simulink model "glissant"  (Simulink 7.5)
settings: Solver=ode45  StartTime=0.0  StopTime=10  RelTol=1e-3

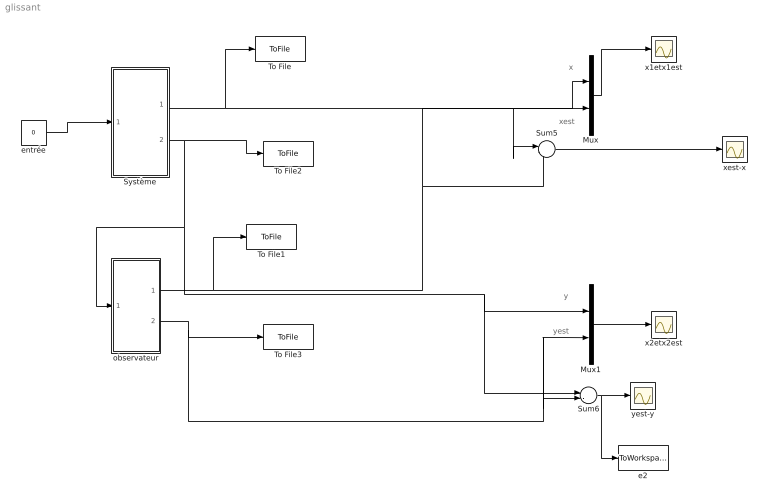
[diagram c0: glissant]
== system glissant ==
  note: x
  note: xest
  note: y
  note: yest
  Mux : Mux  Inputs=2
  Mux1 : Mux  Inputs=2
  Sum5 : Sum  Inputs=|-+  OutDataType=sfix(16)  OutScaling=2^0
  Sum6 : Sum  Inputs=|-+  OutDataType=sfix(16)  OutScaling=2^0
  Système : Subsystem
  To File : ToFile  Filename=x1.mat
  To File1 : ToFile  Filename=x1est.mat
  To File2 : ToFile  Filename=x2.mat
  To File3 : ToFile  Filename=x2est.mat
  e2 : ToWorkspace  VariableName=y  SampleTime=-1  SaveFormat=Array
  entrée : Constant  Value=0  OutDataType=fixdt(1, 16)  OutScaling=2^0
  observateur : Subsystem
  x1etx1est : Scope
  x2etx2est : Scope
  xest-x : Scope
  yest-y : Scope
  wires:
  Mux/1 -> x1etx1est/1
  Sum6/1 -> yest-y/1, e2/1
  Sum5/1 -> xest-x/1
  entrée/1 -> Système/1(u)
  Système/1("x1 ") -> Mux/1, Sum5/1, To File/1
  Système/2("x2 ") -> observateur/1(y), Mux1/1, Sum6/1, To File2/1
  observateur/1("x1 ") -> Sum5/2, Mux/2, To File1/1
  observateur/2("yest ") -> Sum6/2, Mux1/2, To File3/1
  Mux1/1 -> x2etx2est/1

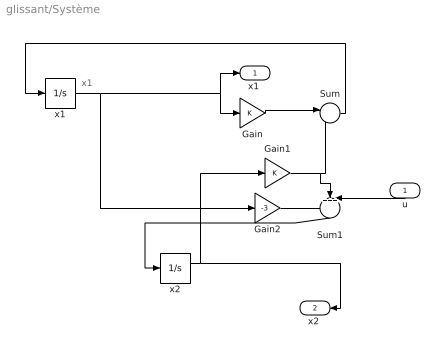
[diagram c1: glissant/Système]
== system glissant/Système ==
  note: x1
  u : Inport
  Gain : Gain  ParameterDataType=fixdt(1, 16)  ParameterScaling=2^0  OutDataType=fixdt(1, 16)  OutScaling=2^0
  Gain1 : Gain  ParameterDataType=fixdt(1, 16)  ParameterScaling=2^0  OutDataType=fixdt(1, 16)  OutScaling=2^0
  Gain2 : Gain  Gain=-3  ParameterDataType=fixdt(1, 16)  ParameterScaling=2^0  OutDataType=fixdt(1, 16)  OutScaling=2^0
  Sum : Sum  Inputs=|-+  OutDataType=sfix(16)  OutScaling=2^0
  Sum1 : Sum  Inputs=+++  OutDataType=sfix(16)  OutScaling=2^0
  x1 : Integrator  InitialCondition=0.5
  x2 : Integrator  InitialCondition=0.5
  "x1 " : Outport
  "x2 " : Outport  Port=2
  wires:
  x1/1 -> Gain/1, "x1 "/1, Gain2/1
  x2/1 -> Gain1/1, "x2 "/1
  Sum/1 -> x1/1
  Sum1/1 -> x2/1
  Gain/1 -> Sum/1
  Gain1/1 -> Sum/2, Sum1/2
  u/1 -> Sum1/3
  Gain2/1 -> Sum1/1

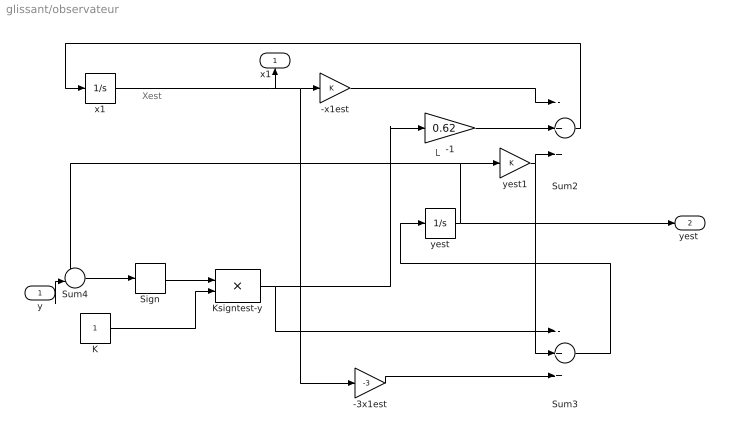
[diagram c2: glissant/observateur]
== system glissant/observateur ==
  note: Xest
  note: L
  y : Inport
  -1 : Gain  Gain=0.62  ParameterDataType=fixdt(1, 16)  ParameterScaling=2^0  OutDataType=fixdt(1, 16)  OutScaling=2^0
  -3x1est : Gain  Gain=-3  ParameterDataType=fixdt(1, 16)  ParameterScaling=2^0  OutDataType=fixdt(1, 16)  OutScaling=2^0
  -x1est : Gain  ParameterDataType=fixdt(1, 16)  ParameterScaling=2^0  OutDataType=fixdt(1, 16)  OutScaling=2^0
  K : Constant  OutDataType=sfix(16)  OutScaling=2^0
  Ksigntest-y : Product  OutDataType=sfix(16)  OutScaling=2^0
  Sign : Signum  ZeroCross=off
  Sum2 : Sum  Inputs=-++  OutDataType=sfix(16)  OutScaling=2^0
  Sum3 : Sum  Inputs=-++  OutDataType=sfix(16)  OutScaling=2^0
  Sum4 : Sum  Inputs=+-  OutDataType=sfix(16)  OutScaling=2^0
  x1 : Integrator
  yest : Integrator
  yest1 : Gain  ParameterDataType=fixdt(1, 16)  ParameterScaling=2^0  OutDataType=fixdt(1, 16)  OutScaling=2^0
  "x1 " : Outport
  "yest " : Outport  Port=2
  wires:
  yest/1 -> Sum4/1, yest1/1, "yest "/1
  -3x1est/1 -> Sum3/3
  Sum4/1 -> Sign/1
  Sign/1 -> Ksigntest-y/1
  K/1 -> Ksigntest-y/2
  Sum2/1 -> x1/1
  Sum3/1 -> yest/1
  x1/1 -> -x1est/1, -3x1est/1, "x1 "/1
  Ksigntest-y/1 -> Sum3/1, -1/1
  -x1est/1 -> Sum2/1
  yest1/1 -> Sum2/3, Sum3/2
  y/1 -> Sum4/2
  -1/1 -> Sum2/2
